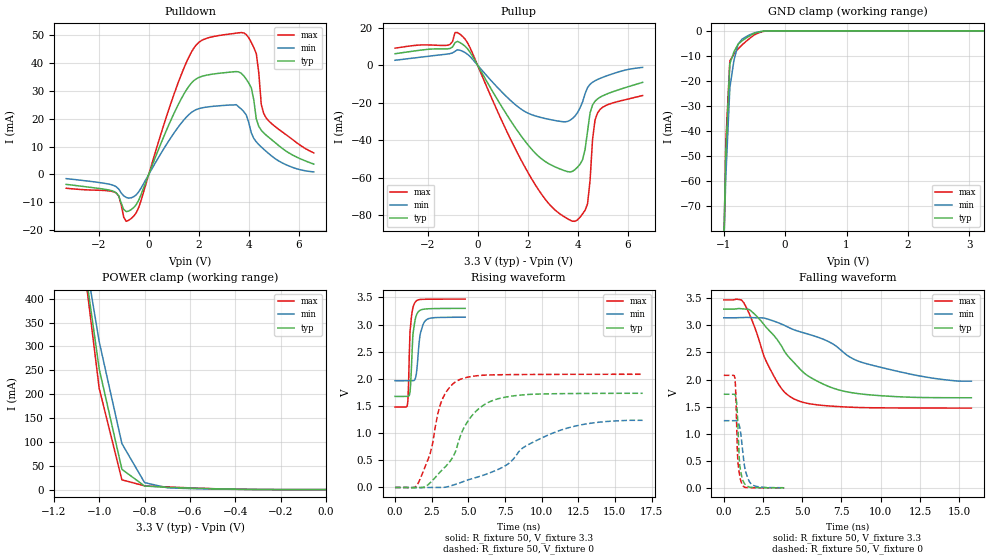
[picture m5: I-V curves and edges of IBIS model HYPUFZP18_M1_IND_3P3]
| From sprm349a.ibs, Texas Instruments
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|   Model Cell HYPUFZP18_M1_IND_3P3
[Model]   HYPUFZP18_M1_IND_3P3
Model_type   I/O
Polarity   Non-Inverting
Enable   Active-Low
Vinl =  0.8V
Vinh =  2V
Cref =  15.0000pF
Rref =  100.0000M
Vref =  0V
Vmeas =  1.65
C_comp   1.500963p   1.465915p   1.537982p
[Model Spec]
Vinl   0.8V   0.8V   0.8V
Vinh   2V   2V   2V
[Temperature Range]   25   125   -40
[Voltage Range]   3.3   3.14   3.47
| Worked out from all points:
|   slope of the pulldown table from 0 to 0.495 V, typ, clamps not added: 44 ohm
|   slope of the pullup table from 0 to 0.495 V, typ, clamps not added: 42.8 ohm
|   GND clamp passes 1 mA (typ) near -0.50 V on its own axis
|   POWER clamp passes 1 mA (typ) near -0.41 V on its own axis
|   rising waveform, R_fixture 50, V_fixture 3.3: 20-80 % time 217ps typ, 300ps min, 175ps max; typ from 1.68 V to 3.3 V
|   rising waveform, R_fixture 50, V_fixture 0: 20-80 % time 2.16ns typ, 4.4ns min, 1.2ns max; typ from 0 V to 1.74 V
|   falling waveform, R_fixture 50, V_fixture 3.3: 20-80 % time 3.14ns typ, 5.71ns min, 1.76ns max; typ from 3.3 V to 1.66 V
|   falling waveform, R_fixture 50, V_fixture 0: 20-80 % time 192ps typ, 363ps min, 150ps max; typ from 1.73 V to 0.001 V
[POWER_clamp]
|   voltage   I(typ)   I(min)   I(max)
-3.3V     9.961A     8.483A     11.27A
-1.067V   478.8mA    500.9mA    470.3mA
-1.033V   365.9mA    405.4mA    341.2mA
-1V       253mA      310mA      212mA
-900mV    42.53mA    96.46mA    20.46mA
-800mV    7.492mA    14.62mA    7.887mA
-700mV    4.749mA    3.86mA     5.601mA
-400mV    851.5uA    522.8uA    761.4uA
-11.55fV  112.1nA    200.9nA    235.2nA
[Pulldown]
|   voltage   I(typ)   I(min)   I(max)
-3.3V     -3.547mA   -1.486mA   -4.928mA
-1.4V     -6.057mA   -3.93mA    -6.213mA
-900mV    -13.28mA   -8.212mA   -16.76mA
-600mV    -11.85mA   -7.958mA   -14.91mA
1.6V      31.52mA    21.37mA    41.96mA
3V        36.41mA    24.71mA    50mA
3.5V      36.83mA    25mA       50.6mA
4V        32.72mA    18.57mA    48.93mA
4.3V      19.94mA    11.7mA     43.35mA
4.5V      15.84mA    9.852mA    25.09mA
4.6V      14.87mA    9.033mA    21.76mA
6.6V      3.718mA    925.6uA    7.735mA
[Pullup]
|   voltage   I(typ)   I(min)   I(max)
-3.3V     6.065mA    2.586mA    9.02mA
-600mV    11.14mA    7.39mA     15.31mA
2.2V      -45.34mA   -26.58mA   -61.36mA
3V        -53.58mA   -29.27mA   -75.93mA
3.8V      -56.58mA   -28.4mA    -83.16mA
4.2V      -50.4mA    -19.68mA   -79.27mA
4.4V      -35.28mA   -11.98mA   -73.9mA
4.5V      -25.43mA   -10.23mA   -61.46mA
4.6V      -21.24mA   -9.135mA   -39.55mA
4.7V      -19.23mA   -8.329mA   -29.16mA
4.8V      -18mA      -7.666mA   -25.45mA
6.6V      -9.206mA   -1.224mA   -16.21mA
[GND_clamp]
|   voltage   I(typ)   I(min)   I(max)
-3.3V     -13.48A    -11.37A    -15.19A
-1.033V   -124.1mA   -117.5mA   -138.7mA
-966.7mV  -49.36mA   -59.06mA   -45.08mA
-900mV    -13.13mA   -22.73mA   -11.96mA
-833.3mV  -8.422mA   -11.83mA   -9.352mA
-766.7mV  -5.368mA   -5.355mA   -7.235mA
-700mV    -3.962mA   -3.31mA    -5.61mA
-566.7mV  -1.872mA   -1.46mA    -2.81mA
-433.3mV  -496.5uA   -419uA     -816.2uA
-300mV    -30.1uA    -42.64uA   -47.75uA
3.233V    79.91nA    2.437uA    205.4nA
[Ramp]
| variable   typ   min   max
dV/dt_f  0.9905248/3.164362n   0.7575388/6.587516n   1.208211/1.763743n
dV/dt_r   1.047452/2.182911n   0.7636201/4.596286n   1.255968/1.205155n
R_load = 50
[Rising Waveform]
R_fixture = 50
V_fixture = 3.3
V_fixture_min = 3.14
V_fixture_max = 3.47
|   time   V(typ)   V(min)   V(max)
0s        1.677V     1.967V     1.483V
828ps     1.678V     1.967V     1.498V
924ps     1.679V     1.967V     1.894V
1.024ns   1.755V     1.967V     2.874V
1.22ns    2.812V     1.967V     3.309V
1.364ns   3.077V     1.992V     3.409V
1.464ns   3.178V     2.106V     3.439V
1.708ns   3.263V     2.81V      3.463V
2.048ns   3.287V     3.065V     3.467V
4.784ns   3.299V     3.137V     3.47V
[Rising Waveform]
R_fixture = 50
V_fixture = 0
V_fixture_min = 0
V_fixture_max = 0
|   time   V(typ)   V(min)   V(max)
0s        38.06uV    22.56uV    59.71uV
1.548ns   -823uV     -1.626mV   58.71mV
2.408ns   88.82mV    -103.2uV   633.7mV
3.1ns     290.8mV    629.7uV    1.536V
4.304ns   818.8mV    73.7mV     1.974V
5.34ns    1.353V     169.3mV    2.05V
7.064ns   1.636V     336mV      2.076V
8.788ns   1.707V     741.2mV    2.081V
11.37ns   1.729V     1.062V     2.084V
16.89ns   1.735V     1.237V     2.086V
[Falling Waveform]
R_fixture = 50
V_fixture = 3.3
V_fixture_min = 3.14
V_fixture_max = 3.47
|   time   V(typ)   V(min)   V(max)
0s        3.3V       3.14V      3.47V
1.284ns   3.302V     3.145V     3.413V
2.572ns   3.01V      3.134V     2.422V
3.22ns    2.805V     3.075V     2.047V
3.864ns   2.522V     3V         1.769V
4.668ns   2.252V     2.899V     1.616V
5.956ns   1.97V      2.785V     1.532V
7.892ns   1.77V      2.441V     1.492V
11.92ns   1.673V     2.098V     1.474V
15.78ns   1.664V     1.97V      1.473V
[Falling Waveform]
R_fixture = 50
V_fixture = 0
V_fixture_min = 0
V_fixture_max = 0
|   time   V(typ)   V(min)   V(max)
0s        1.728V     1.24V      2.077V
704ps     1.724V     1.241V     2.034V
744ps     1.704V     1.241V     1.888V
820ps     1.569V     1.236V     1.167V
900ps     1.154V     1.213V     468.1mV
1.016ns   415.1mV    1.119V     220.5mV
1.176ns   173mV      754.8mV    57.97mV
1.372ns   58.89mV    320.6mV    9.003mV
1.764ns   9.208mV    68.15mV    2.167mV
3.848ns   915.6uV    3.172mV    139.3uV
